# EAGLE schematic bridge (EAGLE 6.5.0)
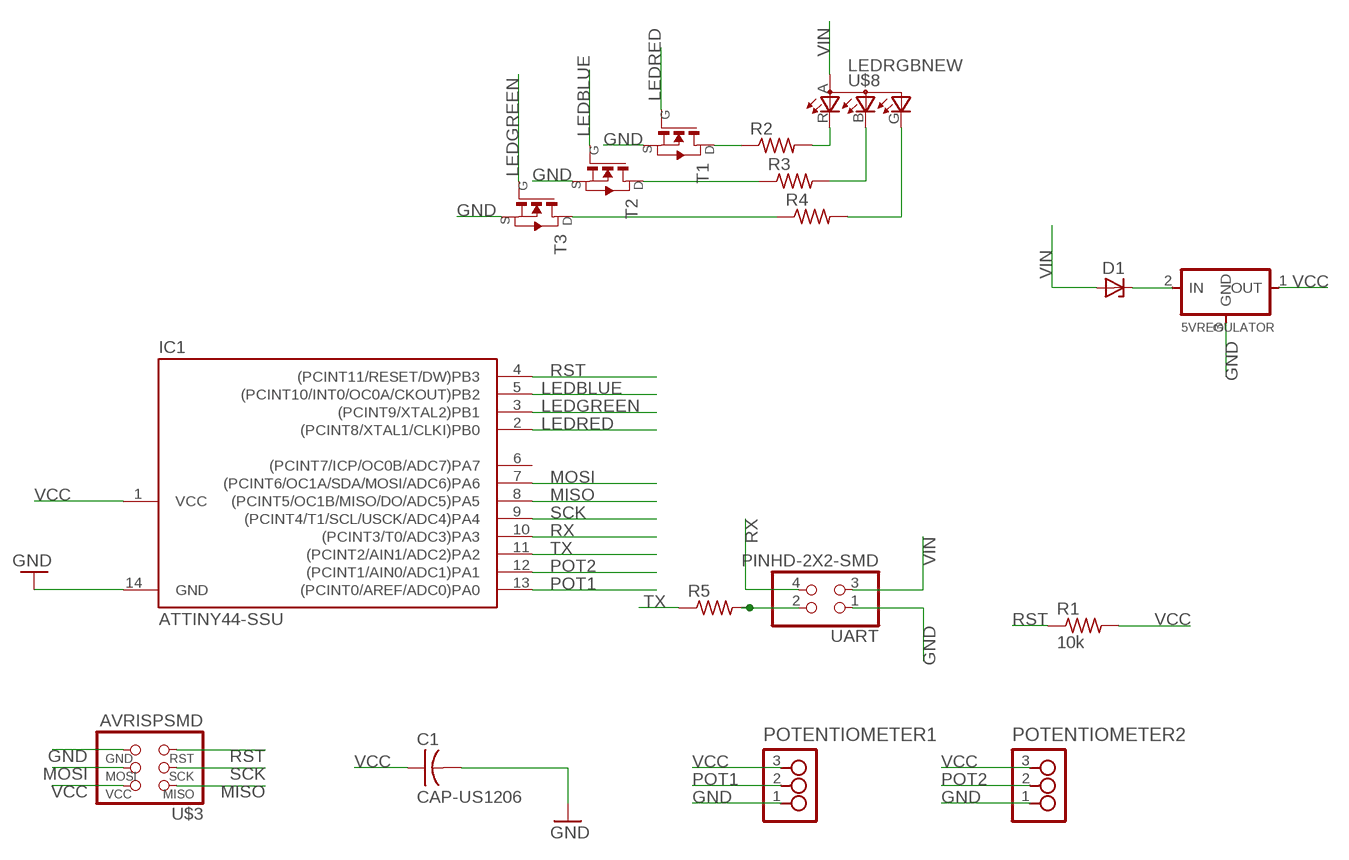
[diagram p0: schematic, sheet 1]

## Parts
5VREGULATOR  REGULATORSOT23  [SOT23]
C1  CAP-US1206  [C1206]
D1  ZENER_DIODESOD123  [SOD123]
IC1  ATTINY44-SSU  [SOIC14]
POTENTIOMETER1  3_PIN_HEADERHEADER  [SMT_PINS_3]
POTENTIOMETER2  3_PIN_HEADERHEADER  [SMT_PINS_3]
R1  10k  RES-US1206  [R1206]
R2  RES-US1206  [R1206]
R3  RES-US1206  [R1206]
R4  RES-US1206  [R1206]
R5  RES-US1206  [R1206]
T1  NMOSFETSOT23  [SOT-23]
T2  NMOSFETSOT23  [SOT-23]
T3  NMOSFETSOT23  [SOT-23]
U$3  AVRISPSMD  [2X03SMD]
U$8  LEDRGBNEW  [P-LCC-4]
UART  PINHD-2X2-SMD  [2X02SMD]

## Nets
GND: 5VREGULATOR.3(GND) C1.2 IC1.14(GND) POTENTIOMETER1.1 POTENTIOMETER2.1 T1.2(S) T2.2(S) T3.2(S) U$3.6(GND) UART.1
LEDBLUE: IC1.5((PCINT10/INT0/OC0A/CKOUT)PB2) T2.3(G)
LEDGREEN: IC1.3((PCINT9/XTAL2)PB1) T3.3(G)
LEDRED: IC1.2((PCINT8/XTAL1/CLKI)PB0) T1.3(G)
MISO: IC1.8((PCINT5/OC1B/MISO/DO/ADC5)PA5) U$3.1(MISO)
MOSI: IC1.7((PCINT6/OC1A/SDA/MOSI/ADC6)PA6) U$3.4(MOSI)
N$1: R2.2 U$8.R(CRED)
N$2: R3.1 T2.1(D)
N$3: R4.1 T3.1(D)
N$4: R2.1 T1.1(D)
N$5: 5VREGULATOR.2(IN) D1.CATHODE
N$6: R5.2 UART.2
N$8: R3.2 U$8.B(CBLUE)
N$9: R4.2 U$8.G(CGREEN)
POT1: IC1.13((PCINT0/AREF/ADC0)PA0) POTENTIOMETER1.2
POT2: IC1.12((PCINT1/AIN0/ADC1)PA1) POTENTIOMETER2.2
RST: IC1.4((PCINT11/RESET/DW)PB3) R1.1 U$3.5(RST)
RX: IC1.10((PCINT3/T0/ADC3)PA3) UART.4
SCK: IC1.9((PCINT4/T1/SCL/USCK/ADC4)PA4) U$3.3(SCK)
TX: IC1.11((PCINT2/AIN1/ADC2)PA2) R5.1
VCC: 5VREGULATOR.1(OUT) C1.1 IC1.1(VCC) POTENTIOMETER1.3 POTENTIOMETER2.3 R1.2 U$3.2(VCC)
VIN: D1.ANODE U$8.A(A2) UART.3
Unconnected: IC1.6((PCINT7/ICP/OC0B/ADC7)PA7)

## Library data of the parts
5VREGULATOR = 01_fab:REGULATOR
C1 = fab:CAP-US
D1 = 01_fab:ZENER_DIODE: zener diode
IC1 = 01_fab:ATTINY44
POTENTIOMETER1 POTENTIOMETER2 = 01_ng:3_PIN_HEADER: 3 SMT pin pads
R1-R5 = fab:RES-US: Resistor (US Symbol)
T1-T3 = 01_fab:NMOSFET: MOS FET
U$3 = fab:AVRISP
U$8 = Juanes Library:LEDRGBNEW
UART = 01_fab:PINHD-2X2-SMD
